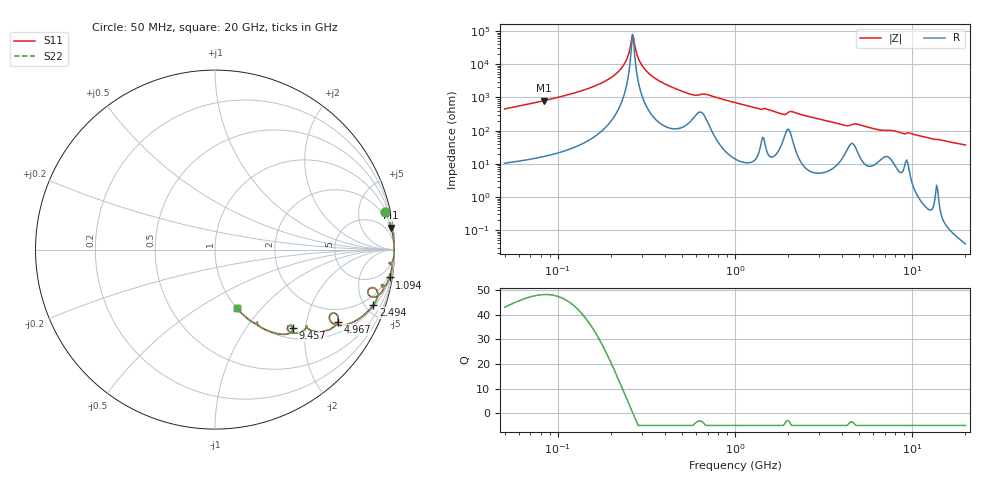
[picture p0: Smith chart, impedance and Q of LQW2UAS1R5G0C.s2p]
!Murata Part Number: LQW2UAS1R5G0C
!These Parameters are Measured in Series Mode Connection
!  o--[Z]--o
!Port1  Port2
!  o-------o
!Freq. Start=50[MHz] Stop=20[GHz], 401[Steps]
# Hz S RI R 50
!Freq.(Hz) S11(Real) S11(Imag) S21(Real) S21(Imag) S12(Real) S12(Imag) S22(Real) S22(Imag)
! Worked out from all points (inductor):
!   401 points, 50 MHz to 20 GHz, reference 50 ohm
!   read as one part in series: L = 1.38 uH near 51.52 MHz
!   highest Q = 48.1 at 83.2 MHz (marker M1), where L = 1.53 uH
!   self-resonance near 263.7 MHz
!   S11 on the Smith chart (normalised r, x): 50 MHz: 1.21, +9.03; 1.094 GHz: 1, -12; 2.494 GHz: 1.15, -5.65; 4.967 GHz: 1.41, -3.06; 9.457 GHz: 1.21, -1.72; 20 GHz: 1.00, -0.74
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5e7  0.9489 0.209  0.0511 -0.209  0.0511 -0.209  0.9489 0.209
8.320417e7  0.9822 0.1224  0.0178 -0.1224  0.0178 -0.1224  0.9822 0.1224
1.364002e8  0.9946 0.0619  0.00539 -0.0619  0.00539 -0.0619  0.9946 0.0619
1.813063e8  0.9976 0.0339  0.00243 -0.0339  0.00243 -0.0339  0.9976 0.0339
2.170075e8  0.9985 0.0175  0.00151 -0.0175  0.00151 -0.0175  0.9985 0.0175
2.409965e8  0.9987 0.00824  0.00127 -0.00824  0.00127 -0.00824  0.9987 0.00824
2.636584e8  0.9988 0.000306  0.00123 -0.000306  0.00123 -0.000306  0.9988 0.000306
2.716764e8  0.9988 -0.00234  0.00124 0.00234  0.00124 0.00234  0.9988 -0.00234
2.841629e8  0.9987 -0.00633  0.00131 0.00633  0.00131 0.00633  0.9987 -0.00633
3.017088e8  0.9985 -0.0117  0.00146 0.0117  0.00146 0.0117  0.9985 -0.0117
3.721004e8  0.9973 -0.0312  0.00271 0.0312  0.00271 0.0312  0.9973 -0.0312
5.575697e8  0.9827 -0.0761  0.0173 0.0761  0.0173 0.0761  0.9827 -0.0761
6.87656e8  0.9798 -0.0765  0.0202 0.0765  0.0202 0.0765  0.9798 -0.0765
1e9  0.9775 -0.1388  0.0225 0.1388  0.0225 0.1388  0.9775 -0.1388
1.094034e9  0.9723 -0.1554  0.0277 0.1554  0.0277 0.1554  0.9723 -0.1554
2.493527e9  0.8824 -0.309  0.1176 0.309  0.1176 0.309  0.8824 -0.309
2.728004e9  0.8578 -0.3383  0.1422 0.3383  0.1422 0.3383  0.8578 -0.3383
4.275624e9  0.6421 -0.3972  0.3579 0.3972  0.3579 0.3972  0.6421 -0.3972
4.966507e9  0.6827 -0.4036  0.3173 0.4036  0.3173 0.4036  0.6827 -0.4036
7.442007e9  0.5096 -0.4302  0.4904 0.4302  0.4904 0.4302  0.5096 -0.4302
9.457416e9  0.4352 -0.4383  0.5648 0.4383  0.5648 0.4383  0.4352 -0.4383
2e10  0.1203 -0.3248  0.8797 0.3248  0.8797 0.3248  0.1203 -0.3248
